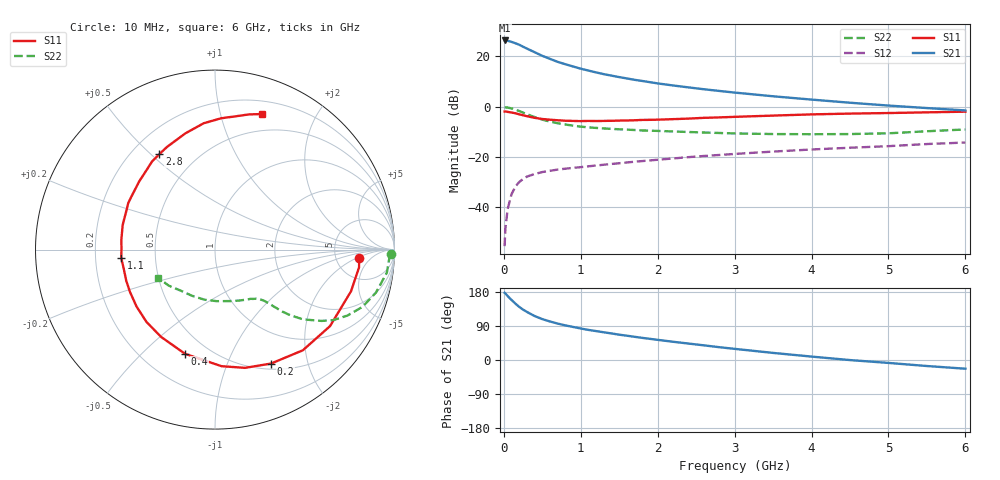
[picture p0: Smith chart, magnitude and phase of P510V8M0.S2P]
! SIEMENS Small Signal Semiconductors
! BFP183
! Si NPN RF Bipolar Junction Transistor in SOT143
! VCE = 10 V  IC = 8 mA
! Common Emitter S-Parameters:  March  1996
# GHz  S  MA  R  50
!  f  S11  S21  S12  S22
! GHz  MAG  ANG  MAG  ANG  MAG  ANG  MAG  ANG
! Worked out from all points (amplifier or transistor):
!   36 points, 10 MHz to 6 GHz, reference 50 ohm
!   highest |S21| = 26.4 dB at 10 MHz (marker M1)
!   |S21| within 3 dB of that: start of sweep to 284.7 MHz
!   unconditionally stable (mu >= 1): 1.424 GHz to 5.745 GHz
!   at 250 MHz: K = 0.26, MSG = 26.3 dB, |S12| = -28.7 dB
!   at 1.4 GHz: K = 0.99, MSG = 17.5 dB, |S12| = -22.7 dB
!   at 6 GHz: K = 0.97, MSG = 6.4 dB, |S12| = -14.2 dB
!   S11 on the Smith chart (normalised r, x): 10 MHz: 8.63, -2.27; 200 MHz: 0.57, -1.45; 400 MHz: 0.37, -0.68; 1.1 GHz: 0.31, -0.04; 2.8 GHz: 0.31, +0.53; 6 GHz: 0.32, +1.36
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0.01  0.8045 -3.3  20.82 177.3  0.0017 77.0  0.9802 -1.5
0.02  0.8087 -7.0  20.71 175.6  0.0038 81.3  0.9722 -3.0
0.05  0.7925 -17.1  20.48 168.7  0.0094 83.9  0.9663 -7.6
0.1  0.7698 -33.6  19.49 158.5  0.0183 71.2  0.9285 -14.9
0.15  0.7445 -48.9  18.32 148.8  0.026 65.5  0.8817 -21.2
0.2  0.7075 -63.8  17.12 140.2  0.032 60.1  0.824 -26.5
0.25  0.6797 -75.8  15.63 132.9  0.0367 55.0  0.7673 -30.8
0.3  0.6506 -86.8  14.36 126.9  0.041 51.2  0.7143 -33.8
0.4  0.6042 -106.0  12.16 116.0  0.0461 45.7  0.6257 -38.4
0.5  0.5717 -121.7  10.3 107.9  0.0505 41.8  0.5559 -41.1
0.6  0.555 -133.5  8.967 101.6  0.0536 40.0  0.5077 -42.7
0.7  0.5401 -144.0  7.819 96.1  0.0565 38.8  0.4717 -43.6
0.9  0.5241 -160.7  6.326 87.2  0.0612 37.6  0.4218 -45.1
1.1  0.5244 -174.9  5.249 79.4  0.0657 37.5  0.3902 -46.5
1.5  0.5323 165.1  3.893 66.8  0.0756 37.9  0.3573 -50.0
1.8  0.5485 151.8  3.26 58.4  0.0835 38.3  0.3389 -53.9
2.2  0.5684 137.9  2.654 48.1  0.0941 37.4  0.3235 -60.1
2.8  0.6155 120.3  2.067 33.8  0.1103 35.2  0.3018 -71.7
3.5  0.6688 104.2  1.618 18.7  0.1289 31.9  0.2875 -88.1
4.5  0.7329 87.2  1.205 -0.2  0.1537 25.7  0.2874 -116.6
5.5  0.7762 76.0  0.944 -15.9  0.182 19.9  0.3266 -142.1
6  0.8002 70.7  0.847 -23.0  0.1951 15.9  0.3548 -153.9
